(* Logix 5000 AddOnInstructionDefinition export Banner_K50Pro_Compact_Aud_PD_v4; software revision 33.00 *)

TYPE Banner_K50ComAud_Adv_v4 :   // Advanced Process Data information for a Banner K50 Compact Audible.
STRUCT
   Feedback : SINT;   // 0 = Off, 3 = On.
   Volume : SINT;   // 0 = Off, 1 = Low, 2 = Medium, 3 = High.
   Type : SINT;   // 0 = Pulse, 1 = Wobble, 2 = Strobe, 3 = Whoop, 4 = Stcatto, 5 = Siren, 6 = Continuous 1, 7 = Continuous 2, 9 = Jingle, 10 = Melody 1, 11 = Melody 2, 12 = Melody 3, 13 = Custom.
END_STRUCT
END_TYPE

TYPE Banner_K50ComAud_MC_v4 :   // Process Data for Multicolor.
STRUCT
   Out_State : SINT;   // Set Output State. 0 = State 1, 1 = State 2, 2 = State 3, 3 = State 4
END_STRUCT
END_TYPE

TYPE Banner_K50ComAud_PDO_v4 :   // UDT that records the converted prcoess data.
STRUCT
   MultiColor : Banner_K50ComAud_MC_v4;   // Only active when Operation Mode set to 0. State tells the light which of the four states it should be in. 0 = State 1, 1 = State 2, 2 = State 3, 3 = State 4.
   Advanced : Banner_K50ComAud_Adv_v4;   // Only active when Operation Mode set to 2.
   OutputByte : SINT;
END_STRUCT
END_TYPE

ADD_ON_INSTRUCTION Banner_K50Pro_Compact_Aud_PD_v4   (* revision 4.0, vendor Banner Engineering *)
// Takes the raw SINT information and converts that data into actual information.
VAR_IN_OUT
   PD : Banner_K50ComAud_PDO_v4; {required}
END_VAR
VAR_INPUT
   Operation_Mode : SINT; {required}   // Linked from Parameters AOI or entered manually.
END_VAR

ROUTINE Logic   (* ladder *)
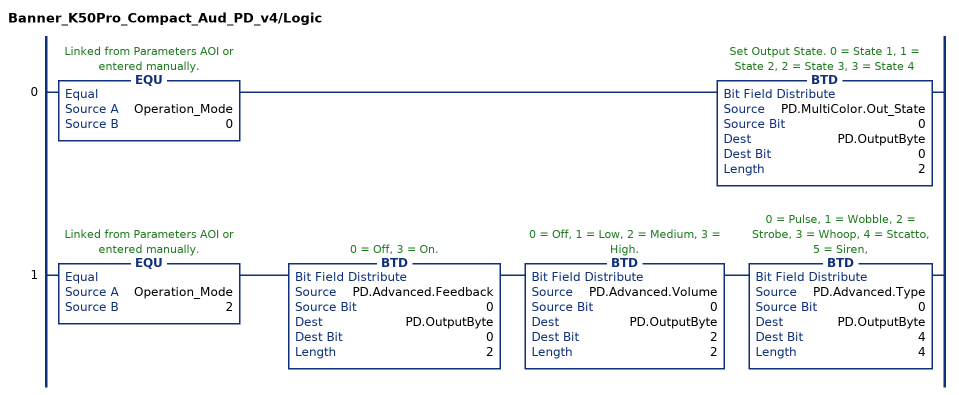
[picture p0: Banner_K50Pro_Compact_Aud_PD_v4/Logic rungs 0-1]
   0: EQU(Operation_Mode,0)BTD(PD.MultiColor.Out_State,0,PD.OutputByte,0,2);
   1: EQU(Operation_Mode,2)BTD(PD.Advanced.Feedback,0,PD.OutputByte,0,2)BTD(PD.Advanced.Volume,0,PD.OutputByte,2,2)BTD(PD.Advanced.Type,0,PD.OutputByte,4,4);
END_ROUTINE
END_ADD_ON_INSTRUCTION
